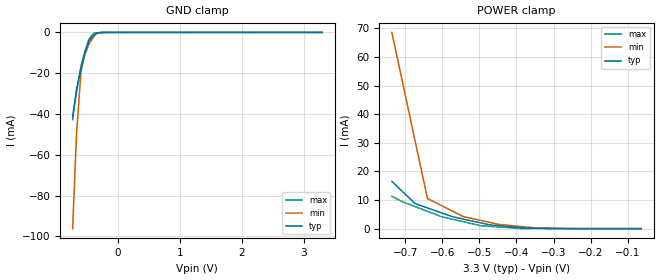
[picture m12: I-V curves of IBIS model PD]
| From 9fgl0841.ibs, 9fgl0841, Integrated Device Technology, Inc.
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[Model]   PD
Model_type   Input
Polarity   Non-Inverting
Vinl = 0.8V
Vinh = 2.0V
|   typ   min   max
C_comp   2pF   1.5pF   2.5pF
|   typ   min   max
[Voltage range]   3.3V   3.135V   3.465V
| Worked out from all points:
|   GND clamp passes 1 mA (typ) near -0.38 V on its own axis
|   POWER clamp passes 1 mA (typ) near -0.45 V on its own axis
[GND_clamp]
|Voltage   I (typ)   I (min)   I (max)
|Note, modeling breaks down at 250mA and above.  This is well beyond the functional   |
|operating range of the device.  Should this scenario occur, catastrophic failure and   |
|possible damage to the device and/or board is of higher concern than the I-V curve   |
|behavior.  The IBIS checker will flag currents in excess of 10A with warnings.  Lines   |
|with currents in excess of 0.35 A have been commented out.  The points still remain|
|available to the user if the user desires to use them.   |
|-3.35893e+00   -1.17049e+02   -9.76985e+01   -1.39583e+02
|-3.25286e+00   -1.14766e+02   -9.76985e+01   -1.33399e+02
|-3.14679e+00   -1.09628e+02   -9.76985e+01   -1.27215e+02
|-3.09796e+00   -1.07263e+02   -9.61466e+01   -1.24368e+02
|-3.03903e+00   -1.04408e+02   -9.36776e+01   -1.20933e+02
|-2.94306e+00   -9.97595e+01   -8.96564e+01   -1.15338e+02
|-2.89592e+00   -9.74758e+01   -8.76810e+01   -1.12589e+02
|-2.82857e+00   -9.42132e+01   -8.48590e+01   -1.08662e+02
|-2.75112e+00   -9.04611e+01   -8.16136e+01   -1.04147e+02
|-2.69388e+00   -8.76878e+01   -7.92146e+01   -1.00809e+02
|-2.61643e+00   -8.39355e+01   -7.59689e+01   -9.62930e+01
|-2.55918e+00   -8.11620e+01   -7.35698e+01   -9.29550e+01
|-2.49184e+00   -7.78989e+01   -7.07472e+01   -8.90280e+01
|-2.40429e+00   -7.36568e+01   -6.70777e+01   -8.39228e+01
|-2.36724e+00   -7.18619e+01   -6.55252e+01   -8.17628e+01
|-2.28980e+00   -6.81091e+01   -6.22789e+01   -7.72464e+01
|-2.19214e+00   -6.33770e+01   -5.81855e+01   -7.15517e+01
|-2.17531e+00   -6.25611e+01   -5.74797e+01   -7.05698e+01
|-2.08607e+00   -5.82368e+01   -5.37390e+01   -6.53659e+01
|-1.98673e+00   -5.34227e+01   -4.95746e+01   -5.95726e+01
|-1.98000e+00   -5.30963e+01   -4.92923e+01   -5.91798e+01
|-1.88571e+00   -4.85268e+01   -4.53394e+01   -5.36810e+01
|-1.79143e+00   -4.39571e+01   -4.13864e+01   -4.81820e+01
|-1.76786e+00   -4.28147e+01   -4.03981e+01   -4.68072e+01
|-1.68367e+00   -3.87345e+01   -3.68684e+01   -4.18972e+01
|-1.59949e+00   -3.46541e+01   -3.33386e+01   -3.69871e+01
|-1.55571e+00   -3.25322e+01   -3.15030e+01   -3.44339e+01
|-1.48163e+00   -2.89414e+01   -2.83967e+01   -3.01129e+01
|-1.40755e+00   -2.53504e+01   -2.52903e+01   -2.57918e+01
|-1.34357e+00   -2.22491e+01   -2.26074e+01   -2.20599e+01
|-1.27959e+00   -1.91478e+01   -1.99245e+01   -1.83280e+01
|-1.21561e+00   -1.60464e+01   -1.72416e+01   -1.45960e+01
|-1.13143e+00   -1.19657e+01   -1.37115e+01   -9.68544e+00
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-735.8mV  -42.77mA   -96.25mA   -40.99mA
-673.5mV  -27.97mA   -49.99mA   -29.38mA
-601.1mV  -17.75mA   -19.48mA   -16.75mA
-543.8mV  -10.98mA   -11.34mA   -9.938mA
-471.4mV  -4.089mA   -5.599mA   -3.287mA
-388.9mV  -1.183mA   -1.845mA   -328.6uA
-351.9mV  -439.7uA   -659.7uA   -216.9uA
-159.9mV  -996.6nA   -4.823uA   -71.72nA
3.295V    7.843nA    1.96uA     174.5pA
[Power_clamp]
|Voltage   I (typ)   I (min)   I (max)
|Note, modeling breaks down at 250mA and above.  This is well beyond the functional   |
|operating range of the device.  Should this scenario occur, catastrophic failure and   |
|possible damage to the device and/or board is of higher concern than the I-V curve   |
|behavior.  The IBIS checker will flag currents in excess of 10A with warnings.  Lines   |
|with currents in excess of 0.35 A have been commented out.  The points still remain|
|available to the user if the user desires to use them.   |
|-3.46500e+00   1.49104e+02   1.25463e+02   1.83372e+02
|-3.35893e+00   1.49104e+02   1.25463e+02   1.75562e+02
|-3.30000e+00   1.49104e+02   1.25463e+02   1.71223e+02
|-3.25286e+00   1.46180e+02   1.25463e+02   1.67752e+02
|-3.19898e+00   1.42838e+02   1.25463e+02   1.63785e+02
|-3.14679e+00   1.39601e+02   1.25463e+02   1.59942e+02
|-3.13500e+00   1.38870e+02   1.25463e+02   1.59074e+02
|-3.09796e+00   1.36573e+02   1.23457e+02   1.56347e+02
|-3.04071e+00   1.33022e+02   1.20358e+02   1.52132e+02
|-3.03903e+00   1.32918e+02   1.20267e+02   1.52008e+02
|-2.99694e+00   1.30307e+02   1.17988e+02   1.48909e+02
|-2.94306e+00   1.26965e+02   1.15070e+02   1.44942e+02
|-2.93464e+00   1.26443e+02   1.14614e+02   1.44322e+02
|-2.89592e+00   1.24041e+02   1.12518e+02   1.41471e+02
|-2.84709e+00   1.21013e+02   1.09874e+02   1.37875e+02
|-2.82857e+00   1.19864e+02   1.08871e+02   1.36512e+02
|-2.79490e+00   1.17776e+02   1.07047e+02   1.34032e+02
|-2.75112e+00   1.15061e+02   1.04677e+02   1.30809e+02
|-2.72250e+00   1.13285e+02   1.03127e+02   1.28701e+02
|-2.69388e+00   1.11510e+02   1.01577e+02   1.26594e+02
|-2.65515e+00   1.09108e+02   9.94806e+01   1.23743e+02
|-2.61643e+00   1.06706e+02   9.73837e+01   1.20891e+02
|-2.59286e+00   1.05244e+02   9.61073e+01   1.19156e+02
|-2.55918e+00   1.03155e+02   9.42840e+01   1.16676e+02
|-2.51036e+00   1.00127e+02   9.16401e+01   1.13081e+02
|-2.49184e+00   9.89782e+01   9.06372e+01   1.11717e+02
|-2.46321e+00   9.72029e+01   8.90873e+01   1.09610e+02
|-2.40429e+00   9.35478e+01   8.58964e+01   1.05271e+02
|-2.39082e+00   9.27123e+01   8.51670e+01   1.04279e+02
|-2.36724e+00   9.12503e+01   8.38907e+01   1.02543e+02
|-2.29821e+00   8.69686e+01   8.01527e+01   9.74603e+01
|-2.28980e+00   8.64464e+01   7.96969e+01   9.68404e+01
|-2.27128e+00   8.52977e+01   7.86940e+01   9.54767e+01
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-735.8mV  16.55mA    68.57mA    11.3mA
-707.1mV  12.98mA    51.26mA    9.395mA
-673.5mV  8.775mA    30.9mA     7.729mA
-639.8mV  7.245mA    10.53mA    6.063mA
-601.1mV  5.485mA    7.992mA    4.147mA
-572.4mV  4.184mA    6.114mA    3.295mA
-543.8mV  3.364mA    4.236mA    2.443mA
-495mV    1.967mA    2.835mA    989.6uA
-471.4mV  1.292mA    2.158mA    786uA
-447.9mV  1.031mA    1.482mA    582.5uA
-351.9mV  144.3uA    283.8uA    48.53uA
-63.98mV  12.08nA    171.6nA    400.1pA
